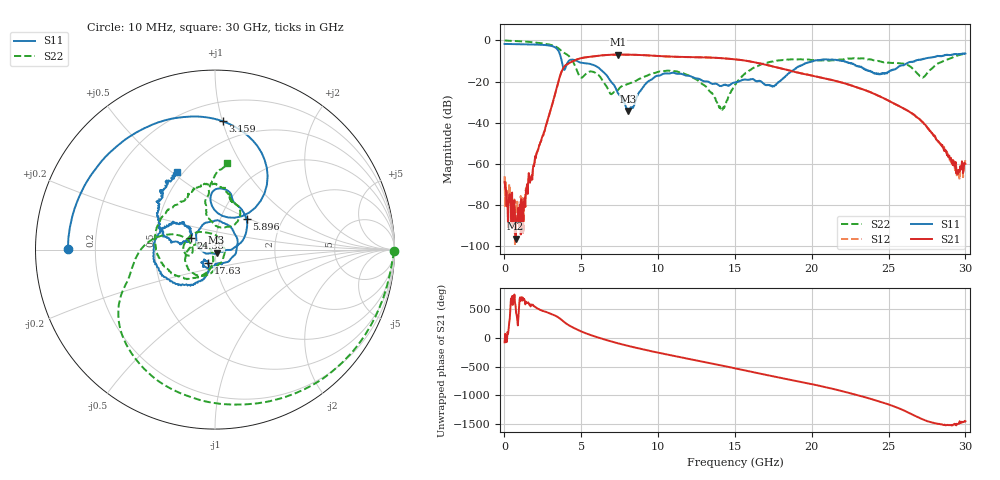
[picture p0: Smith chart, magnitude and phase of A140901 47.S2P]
!  2-Port S-parameters saved by WinCal
! VAR MeasName=S-Parameters (CALIBRATED_DATA) read from VNA (N5244A)
! VAR MeasDate=11/3/2014 9:34:16 AM
! VAR NAME=A140901 47
! VAR FILENAME=A140901 47.S2P
! VAR DATE=11/3/2014 9:34:16 AM
! VAR PHYS_PORTS=1,2
# Hz S RI R 50
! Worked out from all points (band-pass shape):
!   801 points, 10 MHz to 30 GHz, reference 50 ohm
!   highest |S21| = -6.88 dB at 7.395 GHz (marker M1); lowest = -96.4 dB at 722.3 MHz (marker M2)
!   |S21| within 3 dB of the highest: 4.516 GHz to 15.71 GHz (11.2 GHz wide, 111 % of centre)
!   lowest |S11| = -34.3 dB at 8.07 GHz (marker M3), VSWR 1.04, Z = 50.9 - j1.73 ohm
!   |S11| at or under -10 dB: 3.727 GHz to 4.183 GHz (455.1 MHz wide, 11.5 % of centre); 4.716 GHz to 20.12 GHz (15.41 GHz wide, 124 % of centre); 22.09 GHz to 26.72 GHz (4.631 GHz wide, 19 % of centre)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
!   |S22| runs from -33.7 to 0.0 dB; largest |S21 - S12| = 0.0027
!   S11 on the Smith chart (normalised r, x): 10 MHz: 0.10, +0.00; 3.159 GHz: 0.34, +1.00; 5.896 GHz: 1.33, +0.48; 17.63 GHz: 0.92, -0.14; 24.38 GHz: 0.76, +0.10; 30 GHz: 0.47, +0.52
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1e7  -0.8174 0.00182  6.06e-05 -0.000359  0.000227 -0.000444  0.9968 -0.00854
7.222625e8  -0.7809 0.2324  -1.42e-05 -5.27e-06  -3.66e-05 -4.61e-05  0.8617 -0.4333
1.284575e9  -0.6995 0.4015  5.78e-05 -6.79e-05  9.69e-06 -0.000136  0.6366 -0.692
2.296738e9  -0.4238 0.6603  -0.00174 0.00239  -0.00165 0.00246  0.0505 -0.8611
3.15895e9  0.0424 0.7152  0.0251 0.0206  0.025 0.0205  -0.4497 -0.6001
3.871212e9  0.0727 0.1792  0.0165 -0.2249  0.0168 -0.2242  -0.4784 -0.1525
4.471012e9  0.0573 0.335  -0.3135 0.0314  -0.313 0.0306  -0.2879 0.0804
5.033325e9  0.104 0.2654  -0.0928 0.3619  -0.0931 0.3618  -0.1242 -0.00893
5.895538e9  0.1761 0.1691  0.3899 0.1398  0.3897 0.141  -0.153 0.0589
7.395038e9  0.0504 -0.00725  -0.062 -0.4485  -0.0614 -0.448  0.0472 -0.0417
8.069812e9  0.00894 -0.017  -0.3603 -0.2687  -0.3601 -0.2689  0.0155 -0.0869
1.001916e10  -0.0987 0.0992  -0.0694 0.4134  -0.0687 0.4119  -0.0975 -0.1437
1.196851e10  0.1212 0.0672  0.3915 -0.0304  0.3909 -0.0297  -0.1422 0.00895
1.414279e10  0.0152 -0.0781  -0.1979 -0.3126  -0.1975 -0.3145  -0.0205 -0.00956
1.5005e10  -0.00593 -0.0942  -0.3418 -0.0571  -0.3421 -0.057  -0.0141 -0.0822
1.762912e10  -0.0362 -0.0734  0.1645 0.1547  0.1639 0.1553  -0.3139 -0.0437
2.002832e10  -0.2614 -0.1644  0.0102 -0.1387  0.0107 -0.14  -0.2363 0.2336
2.437688e10  -0.1344 0.0661  0.0411 -0.0171  0.0411 -0.017  0.085 0.3009
2.501416e10  -0.1633 0.0441  0.00752 -0.0332  0.00743 -0.0332  0.092 0.2755
2.722592e10  -0.3076 0.1593  0.00923 0.00429  0.00947 0.00457  0.0183 0.1234
2.947518e10  -0.2565 0.3807  0.000328 -0.000567  0.000358 -0.000607  0.00848 0.4278
3e10  -0.2091 0.4306  0.001 -0.00013  0.0012 -0.000223  0.0675 0.4827
